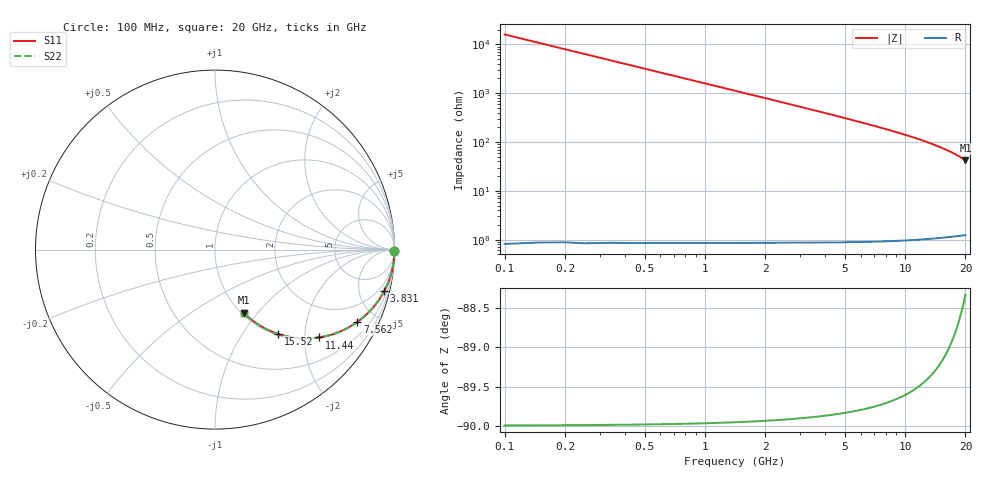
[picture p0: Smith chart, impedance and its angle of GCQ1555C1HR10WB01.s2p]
!Murata Part Number: GCQ1555C1HR10WB01
!These Parameters are Measured in Series Mode Connection
!Data Generated on Mar 13, 2026
!  o--ll--o
!Port1  Port2
!  o------o
!Operation Temp=25[degC], DC Bias Voltage=0[V]
!Freq. Start=100[MHz] Stop=20[GHz] 401[Steps]
# Hz S RI R 50
!Freq.(Hz) S11(Real) S11(Imag) S21(Real) S21(Imag) S12(Real) S12(Imag) S22(Real) S22(Imag)
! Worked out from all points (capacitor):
!   401 points, 100 MHz to 20 GHz, reference 50 ohm
!   read as one part in series: C = 100 fF near 199.5 MHz
!   lowest |Z| = 42.3 ohm at 20 GHz (marker M1)
!   S11 on the Smith chart (normalised r, x): 100 MHz: open; 3.831 GHz: 1.02, -8.16; 7.562 GHz: 1.02, -3.93; 11.44 GHz: 1.02, -2.35; 15.52 GHz: 1.02, -1.47; 20 GHz: 1.02, -0.85
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1e8  1 -0.00628  3.98e-05 0.00628  3.98e-05 0.00628  1 -0.00628
1.4975e8  0.9999 -0.00941  8.93e-05 0.00941  8.93e-05 0.00941  0.9999 -0.00941
2.4925e8  0.9998 -0.0157  0.000247 0.0157  0.000247 0.0157  0.9998 -0.0157
2.99e8  0.9996 -0.0188  0.000356 0.0188  0.000356 0.0188  0.9996 -0.0188
4.4825e8  0.9992 -0.0281  0.0008 0.0281  0.0008 0.0281  0.9992 -0.0281
5.4775e8  0.9988 -0.0344  0.00119 0.0344  0.00119 0.0344  0.9988 -0.0344
6.97e8  0.9981 -0.0437  0.00193 0.0437  0.00193 0.0437  0.9981 -0.0437
9.955e8  0.9961 -0.0624  0.00394 0.0624  0.00394 0.0624  0.9961 -0.0624
1.44325e9  0.9917 -0.0901  0.00826 0.0901  0.00826 0.0901  0.9917 -0.0901
1.9905e9  0.9843 -0.1237  0.0157 0.1237  0.0157 0.1237  0.9843 -0.1237
2.63725e9  0.9726 -0.1625  0.0274 0.1625  0.0274 0.1625  0.9726 -0.1625
3.43325e9  0.954 -0.2086  0.046 0.2086  0.046 0.2086  0.954 -0.2086
3.83125e9  0.943 -0.2309  0.057 0.2309  0.057 0.2309  0.943 -0.2309
5.1745e9  0.898 -0.3012  0.102 0.3012  0.102 0.3012  0.898 -0.3012
6.7665e9  0.831 -0.3727  0.169 0.3727  0.169 0.3727  0.831 -0.3727
7.5625e9  0.7929 -0.4029  0.2071 0.4029  0.2071 0.4029  0.7929 -0.4029
1.005e10  0.6597 -0.4704  0.3403 0.4704  0.3403 0.4704  0.6597 -0.4704
1.1443e10  0.5801 -0.4894  0.4199 0.4894  0.4199 0.4894  0.5801 -0.4894
1.338325e10  0.469 -0.4935  0.531 0.4935  0.531 0.4935  0.469 -0.4935
1.55225e10  0.3531 -0.4705  0.6469 0.4705  0.6469 0.4705  0.3531 -0.4705
1.67165e10  0.2939 -0.4468  0.7061 0.4468  0.7061 0.4468  0.2939 -0.4468
2e10  0.1589 -0.3513  0.8411 0.3513  0.8411 0.3513  0.1589 -0.3513
